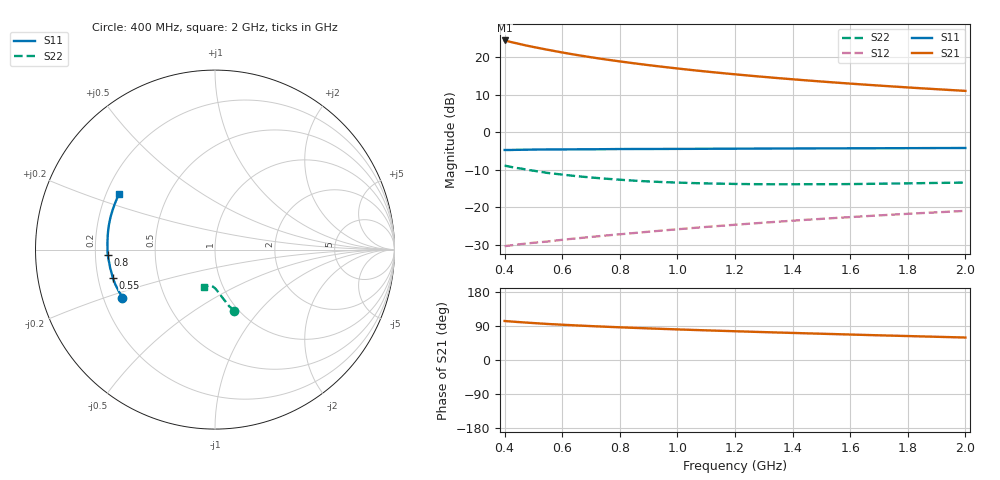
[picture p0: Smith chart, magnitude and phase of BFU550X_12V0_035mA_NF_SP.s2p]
! Filename:  P:\Prog\Test\Noise\ATS_data\Testdata_Net\BFU550X attenuator noise\BFU550X_APG2013_44_C05_12p0V_035mA_NF_CM01_D.sf
! Date/Time: Fri 26/Jul/2013 14:34:25
! BFU550X_APG2013_44_C05_12p0V_1to35mA_NF_CM01_Bias8_R.sf
! Noise Parameter Data File
! BFU550X_APG2013_44_C05_12p0V_1to35mA_NF_CM01
! Date/time: Mon Jul 22 11:28:10 2013
! VAR V_out= 12.001000
! VAR I_out= 35.000000
! VAR V_in= 0.725800
! VAR I_in= 0.340850
! Device data file deembeded for feedlines and parallel
! Original file: \BFU550X attenuator noise\BFU550X_APG2013_44_C05_12p0V_035mA_NF_CM01_R.sf
! Feed-files: PR005V01_100713_Feed1.s2p, PR005V01_100713_Feed2.s2p
! Parallel-file: PR005V01_100713_Par.s2p
# MHz S MA R 50
!  Freq-MHz  S11-mag  S11-arg  S21-mag  S21-arg  S12-mag  S12-arg  S22-mag  S22-arg
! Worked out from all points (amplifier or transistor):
!   37 points, 400 MHz to 2 GHz, reference 50 ohm
!   highest |S21| = 24.5 dB at 400 MHz (marker M1)
!   |S21| within 3 dB of that: start of sweep to 586 MHz
!   unconditionally stable (mu >= 1): 1.314 GHz to end of sweep
!   at 500 MHz: K = 0.71, MSG = 26.1 dB, |S12| = -29.4 dB
!   at 1.1 GHz: K = 0.97, MSG = 20.7 dB, |S12| = -25.2 dB
!   at 2 GHz: K = 1.05, MAG = 14.7 dB, |S12| = -20.9 dB
!   lowest NFmin = 1.41 dB at 460 MHz
!   S11 on the Smith chart (normalised r, x): 400 MHz: 0.28, -0.23; 550 MHz: 0.26, -0.13; 800 MHz: 0.25, -0.02; 2 GHz: 0.25, +0.26
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400  0.5813 -152.6  16.7 102.9  0.03045 49.3  0.3604 -72.7
420  0.5812 -154.4  15.98 101.7  0.03114 49.6  0.3473 -73.9
440  0.5837 -156.2  15.35 100.6  0.03184 49.9  0.3355 -74.6
460  0.585 -157.8  14.74 99.5  0.03251 50.1  0.3274 -75.8
500  0.5885 -161.0  13.67 97.5  0.03377 50.4  0.3081 -77.4
550  0.5909 -164.7  12.54 95.1  0.03516 51.4  0.2873 -79.4
600  0.5909 -167.6  11.55 93.1  0.03701 52.3  0.2734 -81.0
650  0.593 -170.3  10.71 91.2  0.03871 53.0  0.2605 -82.4
700  0.5938 -172.8  9.98 89.5  0.04039 53.8  0.2501 -83.7
750  0.5959 -175.0  9.341 87.8  0.04216 54.4  0.2412 -85.0
800  0.5981 -177.1  8.786 86.3  0.04384 55.0  0.2335 -86.3
850  0.5991 -179.3  8.286 84.8  0.04559 55.7  0.2268 -87.4
900  0.5991 178.9  7.836 83.4  0.04741 56.3  0.2216 -88.5
950  0.6002 177.1  7.438 82.0  0.04928 56.8  0.2173 -89.5
1050  0.6017 173.8  6.742 79.5  0.05301 57.6  0.2109 -91.4
1100  0.6029 172.2  6.441 78.2  0.05493 57.9  0.2086 -92.2
1200  0.6048 169.2  5.914 75.9  0.05871 58.4  0.2052 -94.0
1350  0.6079 165.0  5.264 72.5  0.06451 59.0  0.203 -96.5
1500  0.6104 161.1  4.743 69.3  0.07035 59.2  0.2036 -98.8
1600  0.6117 158.6  4.448 67.2  0.07419 59.3  0.2044 -100.3
1750  0.6138 155.1  4.068 64.2  0.08018 59.2  0.2078 -102.7
2000  0.6181 149.6  3.558 59.3  0.08986 58.8  0.2144 -106.2
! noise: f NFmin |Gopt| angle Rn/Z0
400  1.47  0.3151  -173.9  0.0958
460  1.408  0.3263  -172.1  0.0949
600  1.445  0.3306  -170.9  0.0917
800  1.433  0.3508  -167.4  0.0907
1000  1.471  0.3665  -165.5  0.0861
1200  1.514  0.3782  -160.9  0.0894
1400  1.559  0.3858  -158.6  0.0933
1600  1.592  0.3953  -154.4  0.1024
1800  1.573  0.4365  -154.4  0.0864
2000  1.617  0.4291  -149.1  0.108
